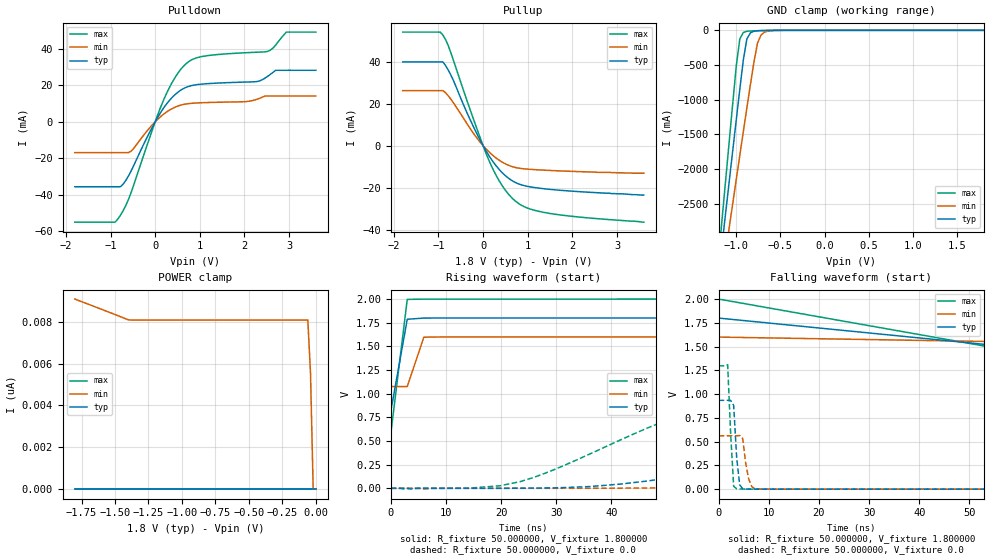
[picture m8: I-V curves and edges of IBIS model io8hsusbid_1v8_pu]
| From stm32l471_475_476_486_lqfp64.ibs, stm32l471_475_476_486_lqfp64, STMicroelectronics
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|   Model io8hsusbid_1v8_pu
[Model]  io8hsusbid_1v8_pu
Model_type I/O
Polarity   Non-Inverting
Enable   Active-Low
Vinl =   0.540000V
Vinh =   1.260000V
Vmeas =  0.900000V
Cref =   100.000000nF
Rref =   1.000000k
Vref =   1.800000V
C_comp   2.022300pF   2.021100pF   2.049600pF
[Temperature Range]   25.000000   0.125000k   -40.000000
[Pullup Reference]   1.800000V   1.600000V   2.000000V
[Pulldown Reference]   0.0V   0.0V   0.0V
[POWER Clamp Reference]   1.800000V   1.600000V   2.000000V
[GND Clamp Reference]   0.0V   0.0V   0.0V
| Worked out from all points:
|   slope of the pulldown table from 0 to 0.27 V, typ, clamps not added: 26.4 ohm
|   slope of the pullup table from 0 to 0.27 V, typ, clamps not added: 30.1 ohm
|   GND clamp passes 1 mA (typ) near -0.60 V on its own axis
|   rising waveform, R_fixture 50.000000, V_fixture 1.800000: 20-80 % time 1.83ns typ, 1.81ns min, 1.81ns max; typ from 0.809 V to 1.8 V
|   rising waveform, R_fixture 50.000000, V_fixture 0.0: 20-80 % time 64.8ns typ, 101ns min, 35.5ns max; typ from 0 V to 0.934 V
|   falling waveform, R_fixture 50.000000, V_fixture 1.800000: 20-80 % time 119ns typ, 161ns min, 92ns max; typ from 1.8 V to 0.809 V
|   falling waveform, R_fixture 50.000000, V_fixture 0.0: 20-80 % time 756ps typ, 988ps min, 727ps max; typ from 0.934 V to 0 V
[Pulldown]
|Voltage   I(typ)   I(min)   I(max)
-1.8V     -35.64mA   -16.93mA   -55.1mA
-840mV    -35.64mA   -16.93mA   -53.52mA
-720mV    -34.31mA   -16.93mA   -48.86mA
-540mV    -27.04mA   -16.13mA   -38.89mA
240mV     9.303mA    5.14mA     14.78mA
480mV     15.67mA    8.374mA    25.64mA
720mV     19.18mA    9.883mA    32.46mA
1.14V     20.87mA    10.54mA    36.19mA
2.28V     22.08mA    12.35mA    38.18mA
2.52V     24.96mA    14.16mA    38.63mA
2.94V     28.27mA    14.16mA    49.23mA
3.6V      28.27mA    14.16mA    49.23mA
[Pullup]
|Voltage   I(typ)   I(min)   I(max)
-1.8V     39.84mA    26.17mA    54.03mA
-960mV    39.84mA    26.17mA    54.03mA
-900mV    39.84mA    26.17mA    52.65mA
-780mV    35.95mA    23.7mA     47.58mA
-240mV    10.08mA    6.588mA    14.1mA
120mV     -4.38mA    -2.702mA   -6.45mA
240mV     -8.143mA   -5.004mA   -12mA
420mV     -12.68mA   -7.723mA   -18.77mA
720mV     -17.48mA   -10.37mA   -26.28mA
1.02V     -19.45mA   -11.2mA    -29.89mA
1.5V      -20.78mA   -11.79mA   -32.25mA
3.6V      -23.5mA    -13.1mA    -36.4mA
[GND_clamp]
|Voltage   I(typ)   I(min)   I(max)
-1.8V     -9.895A    -9.296A    -9.457A
-1.2V     -3.533A    -3.902A    -3.274A
-1.16V    -3.082A    -3.55A     -2.716A
-1.12V    -2.631A    -3.198A    -2.159A
-1.08V    -2.182A    -2.848A    -1.604A
-1V       -1.289A    -2.15A     -512mA
-960mV    -849.4mA   -1.803A    -123.8mA
-920mV    -422.4mA   -1.459A    -30.79mA
-880mV    -123.7mA   -1.118A    -13.63mA
-760mV    -6.32mA    -185mA     -5.692mA
-680mV    -2.569mA   -25.43mA   -2.907mA
1.8V      0A         0A         0A
[POWER_clamp]
|Voltage   I(typ)   I(min)   I(max)
-1.8V     0A         9.088nA    0A
-1.4V     0A         8.095nA    0A
-60mV     0A         8.084nA    0A
-40mV     0A         5.54nA     0A
-20mV     0A         0A         0A
0V        0A         0A         0A
[Ramp]
| variable   typ   min   max
dV/dt_r  0.56065/64.96581n   0.33685/0.11408u   0.77868/35.44838n
dV/dt_f  0.59474/66.70595n   0.31470/0.11610u   0.85906/34.89439n
R_load = 50.000000
[Rising Waveform]
R_fixture= 50.000000
V_fixture= 1.800000
V_fixture_min= 1.600000
V_fixture_max= 2.000000
|time   V(typ)   V(min)   V(max)
0s        808.7mV    1.076V     568.2mV
3.003ns   1.787V     1.076V     1.997V
6.006ns   1.799V     1.597V     1.999V
297.3ns   1.8V       1.6V       2V
[Rising Waveform]
R_fixture= 50.000000
V_fixture= 0.0
V_fixture_min= 0.0
V_fixture_max= 0.0
|time   V(typ)   V(min)   V(max)
0s        2.538nV    69.02nV    1.89nV
23.42ns   1.256mV    -21.35uV   69.76mV
41.44ns   43.88mV    1.561mV    506.3mV
60.66ns   212.9mV    11.95mV    932.7mV
72.67ns   342.9mV    27.96mV    1.098V
88.89ns   509.9mV    66.63mV    1.212V
123.7ns   751.6mV    194.7mV    1.279V
162.8ns   873.8mV    336.9mV    1.294V
219.2ns   923.4mV    479.9mV    1.298V
299.1ns   934.4mV    561.5mV    1.298V
[Falling Waveform]
R_fixture= 50.000000
V_fixture= 1.800000
V_fixture_min= 1.600000
V_fixture_max= 2.000000
|time   V(typ)   V(min)   V(max)
0s        1.8V       1.6V       2V
150.2ns   1.016V     1.47V      598.1mV
300.3ns   821.9mV    1.139V     569mV
450.5ns   810.1mV    1.088V     568.2mV
750.8ns   808.7mV    1.076V     568.2mV
14.86us   808.7mV    1.076V     568.2mV
[Falling Waveform]
R_fixture= 50.000000
V_fixture= 0.0
V_fixture_min= 0.0
V_fixture_max= 0.0
|time   V(typ)   V(min)   V(max)
0s        934.4mV    561.5mV    1.298V
1.802ns   934.4mV    561.5mV    1.31V
2.402ns   933.6mV    561.5mV    581mV
3.003ns   880.4mV    561.5mV    29.9mV
3.604ns   328.2mV    561.1mV    4.044mV
4.204ns   44.87mV    564.6mV    1.698mV
4.805ns   4.525mV    533.6mV    1.139mV
6.006ns   741.2uV    106.6mV    713.9uV
7.808ns   239.3uV    1.591mV    442.8uV
299.1ns   2.538nV    69.02nV    1.89nV
